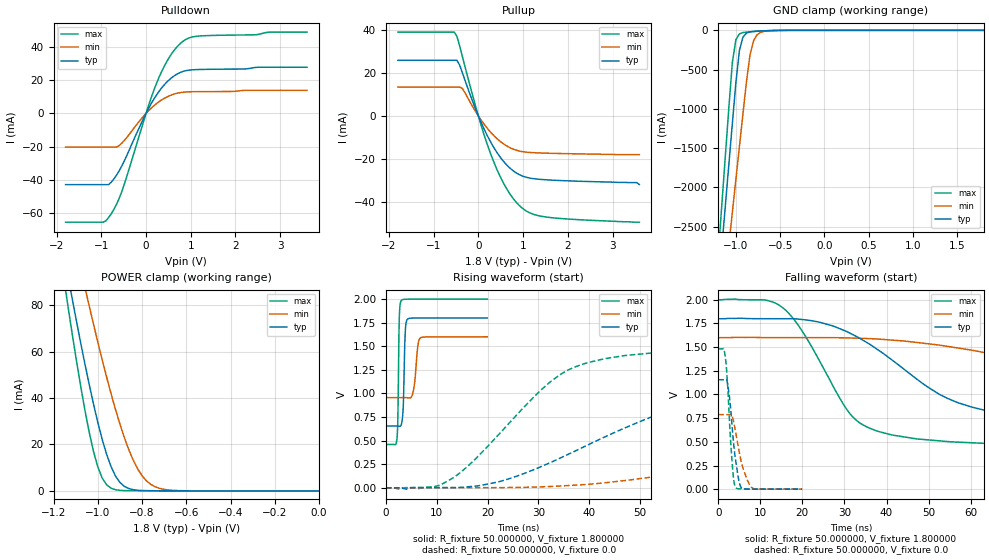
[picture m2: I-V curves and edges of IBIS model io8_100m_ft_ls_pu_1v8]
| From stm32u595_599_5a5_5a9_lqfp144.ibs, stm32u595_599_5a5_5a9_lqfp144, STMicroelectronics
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|   Model io8_100m_ft_ls_pu_1v8
[Model]  io8_100m_ft_ls_pu_1v8
Model_type I/O
Polarity   Non-Inverting
Enable   Active-Low
Vinl =   0.540000V
Vinh =   1.260000V
Vmeas =  0.900000V
Cref =   50.000000pF
Rref =   100.000000M
Vref =   0.0V
C_comp   3.148300pF   3.147400pF   3.196500pF
[Temperature Range]   25.000000   0.140000k   -40.000000
[Pullup Reference]   1.800000V   1.600000V   2.000000V
[Pulldown Reference]   0.0V   0.0V   0.0V
[POWER Clamp Reference]   1.800000V   1.600000V   2.000000V
[GND Clamp Reference]   0.0V   0.0V   0.0V
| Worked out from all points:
|   slope of the pulldown table from 0 to 0.27 V, typ, clamps not added: 21.7 ohm
|   slope of the pullup table from 0 to 0.27 V, typ, clamps not added: 22.6 ohm
|   GND clamp passes 1 mA (typ) near -0.51 V on its own axis
|   POWER clamp passes 1 mA (typ) near -0.86 V on its own axis
|   rising waveform, R_fixture 50.000000, V_fixture 1.800000: 20-80 % time 318ps typ, 631ps min, 229ps max; typ from 0.655 V to 1.8 V
|   rising waveform, R_fixture 50.000000, V_fixture 0.0: 20-80 % time 31.3ns typ, 66.8ns min, 16.5ns max; typ from 0.001 V to 1.16 V
|   falling waveform, R_fixture 50.000000, V_fixture 1.800000: 20-80 % time 24.6ns typ, 55.2ns min, 12.3ns max; typ from 1.8 V to 0.655 V
|   falling waveform, R_fixture 50.000000, V_fixture 0.0: 20-80 % time 1.6ns typ, 2.38ns min, 1.18ns max; typ from 1.16 V to 0.001 V
[Pulldown]
|Voltage   I(typ)   I(min)   I(max)
-1.8V     -42.74mA   -20.21mA   -65.25mA
-960mV    -42.74mA   -20.21mA   -65.25mA
-780mV    -41.3mA    -20.21mA   -60.25mA
-660mV    -37mA      -20.2mA    -54.5mA
-540mV    -31.39mA   -17.82mA   -46.65mA
0V        0A         0A         0A
240mV     11.28mA    6.002mA    18.38mA
480mV     19.17mA    10.02mA    31.83mA
780mV     24.67mA    12.5mA     42.21mA
960mV     25.9mA     12.9mA     45.21mA
1.2V      26.29mA    13.01mA    46.37mA
3.6V      27.65mA    13.81mA    48.71mA
[Pullup]
|Voltage   I(typ)   I(min)   I(max)
-1.8V     26.06mA    13.5mA     39.23mA
-540mV    26.06mA    13.5mA     39.23mA
-480mV    26.06mA    13.5mA     37.18mA
-360mV    20.34mA    12.93mA    27.94mA
0V        590fA      222pA      10fA
300mV     -13.1mA    -8.158mA   -19.11mA
480mV     -18.98mA   -11.71mA   -27.97mA
660mV     -23.42mA   -14.29mA   -34.95mA
1.02V     -28.29mA   -16.75mA   -43.65mA
1.26V     -29.33mA   -17.15mA   -46.11mA
1.62V     -29.92mA   -17.41mA   -47.45mA
3.6V      -32mA      -18mA      -49.6mA
[GND_clamp]
|Voltage   I(typ)   I(min)   I(max)
-1.8V     -9.707A    -9.942A    -9.774A
-1.2V     -3.309A    -4.006A    -2.864A
-1.16V    -2.777A    -3.584A    -2.239A
-1.12V    -2.246A    -3.162A    -1.614A
-1.04V    -1.186A    -2.319A    -408.6mA
-1V       -663.9mA   -1.898A    -117.8mA
-960mV    -254mA     -1.478A    -45.14mA
-920mV    -86.03mA   -1.06A     -28.58mA
-840mV    -19.12mA   -308.9mA   -18.74mA
-800mV    -13.39mA   -130.8mA   -15.31mA
-720mV    -7.948mA   -25.37mA   -9.381mA
1.8V      0A         14.97nA    0A
[POWER_clamp]
|Voltage   I(typ)   I(min)   I(max)
-1.8V     470.9mA    433.7mA    554.6mA
-1.14V    95.28mA    122.7mA    82.88mA
-1.12V    85mA       114mA      70.34mA
-1.06V    55.55mA    88.43mA    35.73mA
-1.04V    46.38mA    80.17mA    25.83mA
-1V       29.54mA    64.14mA    10.37mA
-940mV    10.43mA    41.88mA    1.177mA
-900mV    3.66mA     28.79mA    250.5uA
-840mV    527.2uA    13.26mA    95.74uA
-800mV    153.8uA    6.55mA     88.56uA
-740mV    60.02uA    1.742mA    70.74uA
0V        0A         18.15nA    0A
[Ramp]
| variable   typ   min   max
dV/dt_r  0.69287/31.23698n   0.47203/66.69337n   0.88855/16.46443n
dV/dt_f  0.68714/24.55353n   0.38629/55.14762n   0.92439/12.24842n
R_load = 50.000000
[Rising Waveform]
R_fixture= 50.000000
V_fixture= 1.800000
V_fixture_min= 1.600000
V_fixture_max= 2.000000
|time   V(typ)   V(min)   V(max)
0s        654.8mV    956mV      459.3mV
2.202ns   654.6mV    956mV      532.6mV
2.362ns   654.3mV    956mV      757mV
2.643ns   652.1mV    956.1mV    1.8V
3.043ns   671.3mV    956.1mV    1.986V
3.443ns   894.1mV    956.1mV    1.996V
3.844ns   1.678V     955.8mV    1.998V
4.244ns   1.786V     954.5mV    1.999V
6.807ns   1.8V       1.59V      1.999V
19.94ns   1.8V       1.6V       2V
[Rising Waveform]
R_fixture= 50.000000
V_fixture= 0.0
V_fixture_min= 0.0
V_fixture_max= 0.0
|time   V(typ)   V(min)   V(max)
0s        611.3uV    688.3uV    577.8uV
9.61ns    1.985mV    1.54mV     13.31mV
13.61ns   3.167mV    1.564mV    119.8mV
23.22ns   79.37mV    2.589mV    625.6mV
36.04ns   359.9mV    24.73mV    1.253V
53.65ns   780.3mV    124mV      1.435V
68.07ns   994.5mV    244.5mV    1.466V
81.68ns   1.08V      361.4mV    1.476V
153ns     1.153V     714.9mV    1.482V
398.8ns   1.155V     787.4mV    1.482V
[Falling Waveform]
R_fixture= 50.000000
V_fixture= 1.800000
V_fixture_min= 1.600000
V_fixture_max= 2.000000
|time   V(typ)   V(min)   V(max)
0s        1.8V       1.6V       2V
15.22ns   1.8V       1.6V       1.92V
20.02ns   1.791V     1.6V       1.666V
32.03ns   1.631V     1.596V     760.4mV
37.64ns   1.482V     1.586V     616.2mV
47.25ns   1.16V      1.549V     530.9mV
64.06ns   827.4mV    1.436V     483.3mV
99.3ns    692.3mV    1.146V     462.5mV
171.4ns   657.6mV    992.7mV    459.3mV
398.8ns   654.8mV    956mV      459.3mV
[Falling Waveform]
R_fixture= 50.000000
V_fixture= 0.0
V_fixture_min= 0.0
V_fixture_max= 0.0
|time   V(typ)   V(min)   V(max)
0s        1.155V     787.4mV    1.482V
1.281ns   1.155V     787.4mV    1.486V
1.682ns   1.156V     787.4mV    1.4V
2.402ns   1.067V     787.3mV    972.3mV
3.323ns   654.3mV    774mV      275.5mV
3.724ns   456.5mV    700.9mV    89.25mV
4.084ns   325.5mV    617.5mV    22.72mV
5.285ns   31.71mV    329.5mV    3.445mV
7.888ns   1.04mV     20.57mV    2.271mV
19.94ns   611.3uV    688.3uV    577.8uV
